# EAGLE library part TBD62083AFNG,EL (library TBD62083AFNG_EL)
BiCD Integrated Circuit Silicon Monolithic Source: Datasheet
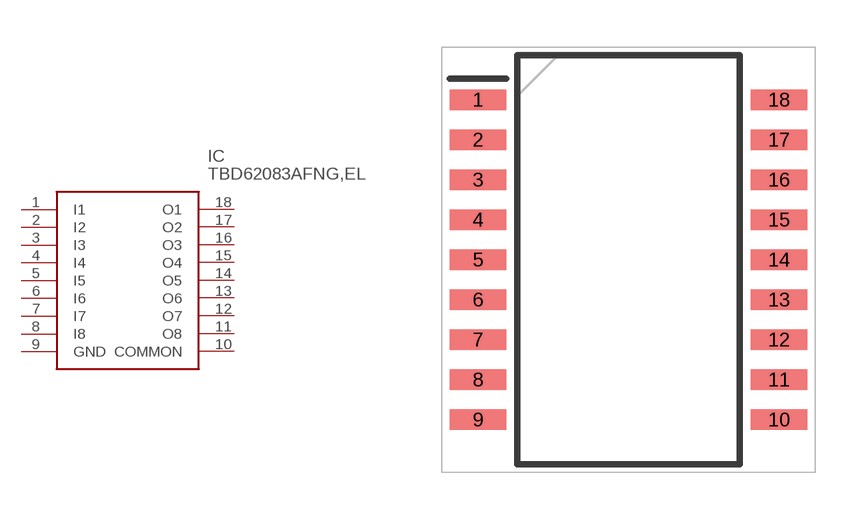
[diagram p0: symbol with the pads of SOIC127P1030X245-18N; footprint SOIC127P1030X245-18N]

Designator prefix IC

## TBD62083AFNG,EL (Description: BiCD Integrated Circuit Silicon Monolithic; Height: 2.45mm; Manufacturer_Name: Toshiba; Manufacturer_Part_Number: TBD62083AFNG,EL; Mouser_Part_Number: 757-TBD62083AFNGEL; Mouser_Price-Stock: https://www.mouser.co.uk/ProductDetail/Toshiba/TBD62083AFNGEL?qs=fSnNYG2PaKLeeuoLxGSskQ%3D%3D)  [SOIC127P1030X245-18N]
1  I1
2  I2
3  I3
4  I4
5  I5
6  I6
7  I7
8  I8
9  GND
10  COMMON
11  O8
12  O7
13  O6
14  O5
15  O4
16  O3
17  O2
18  O1

## Footprint SOIC127P1030X245-18N (pad centres in mm)
SOP18-P-375-1.27
smd 1.8 x 0.65: 1 -4.775,5.08; 2 -4.775,3.81; 3 -4.775,2.54; 4 -4.775,1.27; 5 -4.775,0; 6 -4.775,-1.27; 7 -4.775,-2.54; 8 -4.775,-3.81; 9 -4.775,-5.08; 10 4.775,-5.08; 11 4.775,-3.81; 12 4.775,-2.54; 13 4.775,-1.27; 14 4.775,0; 15 4.775,1.27; 16 4.775,2.54; 17 4.775,3.81; 18 4.775,5.08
